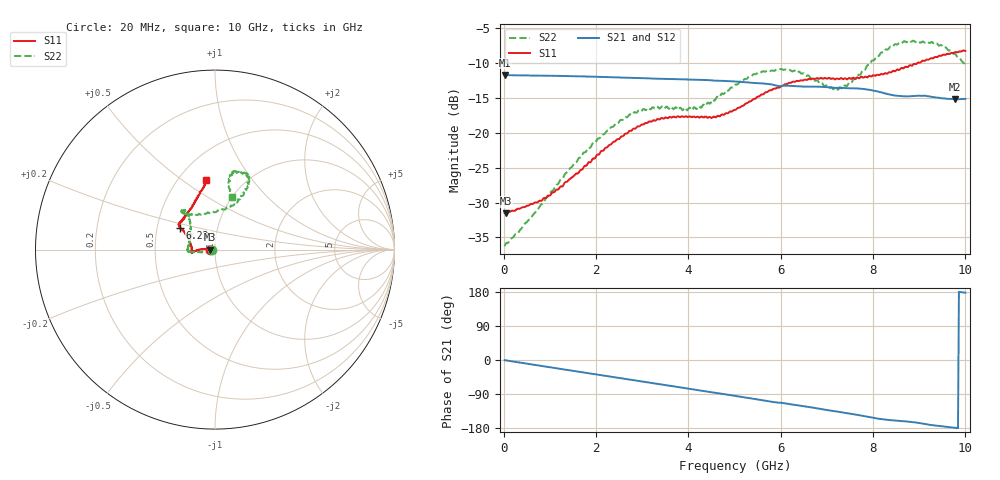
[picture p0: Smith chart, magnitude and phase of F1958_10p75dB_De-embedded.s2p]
! Integrated Device Technology
! Corporate Headquarters
! 6024 Silver Creek Valley Road
! San Jose, CA 95138  USA
! Phone:  1-408-284-8200
! Toll Free:  1-800-223-1366
! Webpage:  http://www.idt.com/
! Timing and RF Division
! 515 Groton Road, Suite 102
! Westford, MA 01886-6024
! Device:  F1958
! Description: 7-bit 0.25 dB Digital Step Attenuator
! Frequency:  0.001 -  6.000 GHz
! Package:  4x4 mm Thin QFN Plastic Package: 24 pin
! Ports:  2 RF, 12 DC
!  Pin  1  = D0
!  Pin  2  = VDD
!  Pin  3  = VMODE
!  Pin  4  = GND
!  Pin  5  = RF1  =  Port 1
!  Pin  6  = GND
!  Pin  7  = GND
!  Pin  8  = GND
!  Pin  9  = GND
!  Pin 10  = GND
!  Pin 11  = GND
!  Pin 12  = GND
!  Pin 13  = GND
!  Pin 14  = RF2  =  Port 2
!  Pin 15  = GND
!  Pin 16  = LE
!  Pin 17  = CLK
!  Pin 18  = DATA
!  Pin 19  = D6
!  Pin 20  = D5
!  Pin 21  = D4
!  Pin 22  = D3
!  Pin 23  = D2
!  Pin 24  = D1
! State:  43
! Atten State:  10.75 dB
! Voltage:  +3.30 Volts
! Current:  0.258 mA
! Data:  The device was measured on a F1958 evaluation board which has
!  individual transmission lines to the RF pins.  Data was collected
!  using a calibrated network analyzer.  The evaluation board was
!  de-embedded using Automatic Fixture Removal (AFR).
!  The reference plane is the edge of the package pin.
! Misc:
!  Action Tracker AT0419
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# GHz S dB R 50
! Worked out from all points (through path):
!   500 points, 20 MHz to 10 GHz, reference 50 ohm
!   highest |S21| = -11.69 dB at 20 MHz (marker M1); lowest = -15.2 dB at 9.78 GHz (marker M2)
!   group delay of S21, straight-line fit = 51.6 ps
!   lowest |S11| = -31.5 dB at 40 MHz (marker M3), VSWR 1.05, Z = 47.4 - j0.0711 ohm
!   |S11| at or under -10 dB: start of sweep to 8.956 GHz
!   |S22| runs from -36.3 to -6.7 dB; largest |S21 - S12| = 0.00089
!   S11 on the Smith chart (normalised r, x): 20 MHz: 0.95, -0.00; 6.22 GHz: 0.66, +0.17; 10 GHz: 0.68, +0.62
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0.02  -31.48 -178.3  -11.69 -0.5  -11.69 -0.5  -36.26 -173.6
0.04  -31.51 -178.4  -11.70 -0.9  -11.69 -0.9  -35.94 -171.0
0.8  -29.75 176.0  -11.78 -15.3  -11.78 -15.3  -30.38 -160.5
1.7  -25.26 177.0  -11.89 -32.3  -11.89 -32.2  -23.19 -168.5
2.6  -20.38 -178.1  -12.07 -49.2  -12.05 -49.2  -17.94 -174.6
2.92  -19.06 -175.2  -12.12 -55.2  -12.11 -55.3  -16.78 -175.3
3.36  -18.06 -172.8  -12.23 -63.5  -12.23 -63.6  -16.43 -177.2
4.22  -17.74 -176.6  -12.38 -79.7  -12.39 -79.8  -16.18 155.5
4.62  -17.61 173.7  -12.50 -87.2  -12.51 -87.3  -14.81 139.8
5.02  -16.69 162.8  -12.61 -94.9  -12.62 -94.9  -13.05 130.3
5.56  -14.61 151.9  -12.89 -105.1  -12.90 -105.1  -11.35 127.7
6.22  -12.79 147.9  -13.25 -116.9  -13.26 -116.9  -11.05 131.9
6.68  -12.23 145.3  -13.36 -125.3  -13.37 -125.3  -12.11 126.2
7.08  -12.22 141.7  -13.47 -133.8  -13.48 -133.6  -13.43 108.3
7.32  -12.15 139.5  -13.54 -138.1  -13.55 -138.0  -13.62 91.8
7.58  -12.08 135.2  -13.61 -143.1  -13.61 -143.0  -12.26 74.4
7.9  -11.90 127.4  -13.79 -150.4  -13.78 -150.4  -10.23 65.5
8.34  -11.31 118.0  -14.46 -158.4  -14.46 -158.5  -7.89 62.6
8.74  -10.57 110.8  -14.75 -162.4  -14.76 -162.3  -6.92 66.3
9.24  -9.31 102.2  -14.79 -171.3  -14.79 -171.3  -7.08 75.2
9.78  -8.39 97.8  -15.17 -179.1  -15.20 -179.1  -8.67 77.3
10  -8.22 97.3  -15.12 177.5  -15.15 177.5  -10.23 72.5
